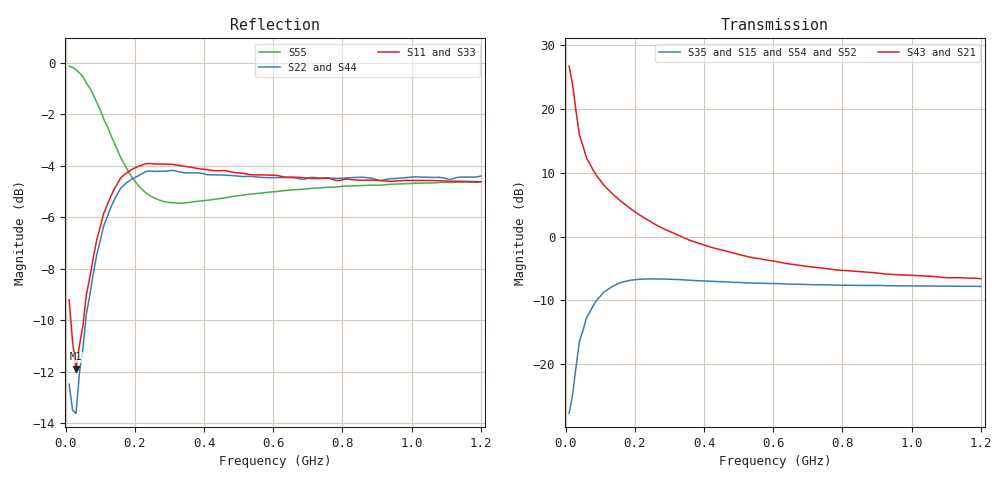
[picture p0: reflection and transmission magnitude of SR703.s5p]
!  POLYFET RF DEVICES
!  S PARAMETERS FOR
!  SR703 (EACH SIDE)
!  VDS=28, IDQ=600MA
! S1A3Die Vds=28Vdc, Idq=600ma, Vgsth=2.63Vdc
! Date: Thu Jul 23 11:57:09 1998
!AWR Design Environment (2053) Wed Feb 04 15:40:52 2004
!freq-unit  param-type  data-format  keyword  impedance-ohms
# MHz  S  MA  R  50
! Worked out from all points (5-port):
!   120 points, 10 MHz to 1.2 GHz, reference 50 ohm
!   strongest paths, dB at 10 MHz, 310 MHz, 610 MHz, 910 MHz, 1.2 GHz:
!     S43: 26.7, 0.6, -3.9, -5.8, -6.6
!     S21: 26.7, 0.6, -3.9, -5.8, -6.6
!     S35: -27.7, -6.7, -7.4, -7.7, -7.8
!     S15: -27.7, -6.7, -7.4, -7.7, -7.8
!     S54: -28.0, -6.8, -7.4, -7.7, -7.8
!     S52: -28.0, -6.8, -7.4, -7.7, -7.8
!   lowest |S11| = -11.9 dB at 30 MHz (marker M1), VSWR 1.68, Z = 48.4 - j25.8 ohm
!   |S11| at or under -10 dB: 14.85 MHz to 51.71 MHz (36.87 MHz wide, 111 % of centre)
